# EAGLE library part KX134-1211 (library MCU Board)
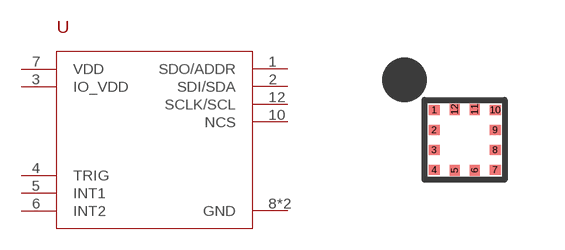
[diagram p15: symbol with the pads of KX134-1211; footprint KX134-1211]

Designator prefix U

## KX134-1211  [KX134-1211]
1  SDO/ADDR
2  SDI/SDA
3  IO_VDD
4  TRIG
5  INT1
6  INT2
7  VDD
8  GND
9  GND
10  NCS
12  SCLK/SCL

## Footprint KX134-1211 (pad centres in mm)
smd 0.275 x 0.25: 1 -0.762,0.75; 2 -0.762,0.25; 3 -0.762,-0.25; 4 -0.762,-0.75; 7 0.762,-0.75; 8 0.762,-0.25; 9 0.762,0.25; 10 0.762,0.75
smd 0.25 x 0.275: 5 -0.25,-0.762; 6 0.25,-0.762; 11 0.25,0.762; 12 -0.25,0.762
